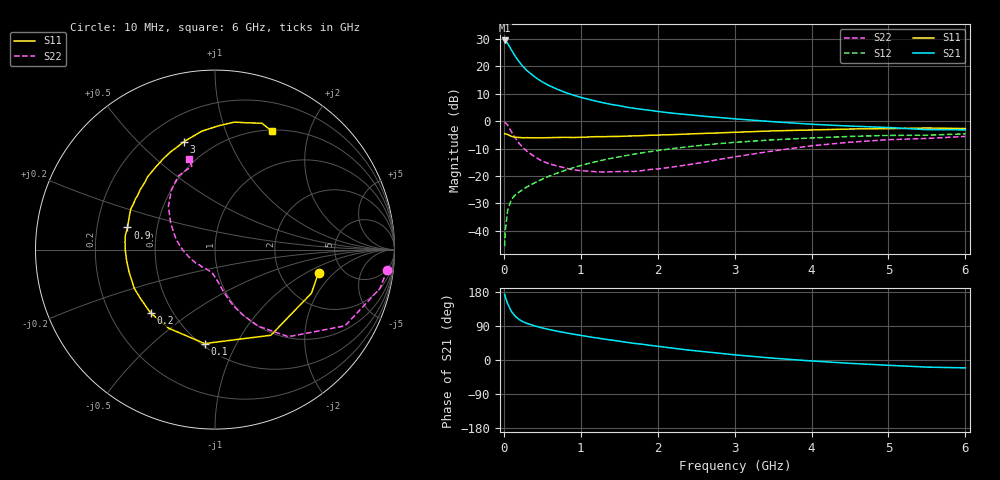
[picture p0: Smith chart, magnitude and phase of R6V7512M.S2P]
! SIEMENS Small Signal Semiconductors
! BFR193
! Si NPN RF Bipolar Junction Transistor in SOT23
! VCE = 0.75 V  IC = 12 mA
! Common Emitter S-Parameters:  May  1996
# GHz  S  MA  R  50
!  f  S11  S21  S12  S22
! GHz  MAG  ANG  MAG  ANG  MAG  ANG  MAG  ANG
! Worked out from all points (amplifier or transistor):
!   36 points, 10 MHz to 6 GHz, reference 50 ohm
!   highest |S21| = 29.5 dB at 10 MHz (marker M1)
!   |S21| within 3 dB of that: start of sweep to 89.5 MHz
!   unconditionally stable (mu >= 1): 631.9 MHz to 2.258 GHz
!   at 250 MHz: K = 0.72, MSG = 22.4 dB, |S12| = -24.9 dB
!   at 1.4 GHz: K = 1.05, MAG = 8.5 dB, |S12| = -13.6 dB
!   at 6 GHz: K = 0.98, MSG = 0.7 dB, |S12| = -4.6 dB
!   S11 on the Smith chart (normalised r, x): 10 MHz: 3.33, -1.31; 100 MHz: 0.52, -0.75; 200 MHz: 0.38, -0.36; 900 MHz: 0.34, +0.11; 3 GHz: 0.35, +0.69; 6 GHz: 0.52, +1.46
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0.01  0.5908 -12.5  29.8 173.2  0.0052 84.9  0.966 -6.7
0.02  0.5898 -24.3  29.11 166.2  0.0104 79.8  0.9446 -13.2
0.05  0.5698 -56.9  26.31 148.3  0.0236 67.8  0.8397 -30.4
0.1  0.5267 -96.3  19.9 127.6  0.0374 56.6  0.6344 -49.9
0.15  0.5085 -120.5  15.18 114.9  0.0454 53.3  0.4895 -60.6
0.2  0.5032 -135.4  12.1 106.7  0.0509 53.1  0.3916 -67.3
0.25  0.4968 -146.0  9.927 100.9  0.0566 53.3  0.3256 -72.1
0.3  0.499 -154.2  8.411 96.6  0.0629 54.9  0.283 -75.0
0.4  0.4948 -165.4  6.463 90.1  0.0746 57.5  0.2236 -79.9
0.5  0.4963 -173.2  5.21 84.6  0.0872 59.0  0.1855 -83.9
0.6  0.4999 -179.7  4.386 80.0  0.1004 60.2  0.1647 -87.3
0.7  0.5034 174.9  3.805 75.7  0.1133 60.6  0.1507 -90.4
0.9  0.5031 165.8  2.997 68.3  0.1412 60.6  0.1291 -98.0
1.1  0.5134 158.2  2.506 61.6  0.1688 59.8  0.1222 -106.5
1.3  0.5209 150.8  2.156 55.3  0.1962 58.1  0.1177 -115.1
1.6  0.534 141.4  1.798 46.5  0.2365 54.8  0.1209 -129.6
2.2  0.5677 125.0  1.394 31.2  0.3164 47.0  0.1457 -159.3
3  0.6262 106.0  1.103 13.6  0.4103 34.6  0.2223 165.8
3.5  0.6638 96.4  0.977 4.8  0.4558 26.7  0.2862 149.5
4.5  0.7186 81.3  0.813 -8.8  0.5258 12.3  0.4125 126.0
5.5  0.751 69.7  0.699 -18.8  0.5542 -1.5  0.4832 105.5
6  0.7321 64.3  0.695 -20.8  0.5869 -5.6  0.5261 105.9
